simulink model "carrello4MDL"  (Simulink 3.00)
settings: Solver=ode45  SolverMode=SingleTasking  StartTime=0.0  StopTime=10.0  RelTol=1e-6  AbsTol=1e-7
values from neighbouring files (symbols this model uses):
  b1 = 2*1500*N/(m/sec)    (= 3000)    [carrello2.M]    (also in carrello3.M; carrello1.M; carrello4.M; carrello5.M)
  b2 = 2*1500*N/(m/sec)    (= 3000)    [carrello2.M]    (also in carrello3.M; carrello1.M; carrello4.M; carrello5.M)
  K = 0.8*1800*N/cm    (= 144000)    [carrello2.M]    (also in carrello3.M; carrello1.M; carrello4.M; carrello5.M)
  Kg = 1    [carrello2.M]    (also in carrello3.M; carrello1.M; carrello4.M = 10000000; carrello5.M)
  Kp = 2*1800*N/cm    (= 360000)    [carrello2.M]    (also in carrello3.M; carrello1.M; carrello4.M; carrello5.M)
  Ma = 3850*Kg    (= 3850)    [carrello2.M]    (also in carrello3.M; carrello1.M; carrello4.M; carrello5.M)
  mr = 2*134*Kg+524*Kg    (= 792)    [carrello2.M]    (also in carrello3.M; carrello1.M; carrello4.M; carrello5.M)
  R = 1    [carrello4.M]    (also in carrello5.M = 0.1; carrello6.M = 0.1)
  t1 = 0    [carrello4.M]
  t2 = 0    [carrello4.M]
  X_12_0 = -Mag/K    (= -0.26228125)    [carrello2.M]    (also in carrello3.M = 0; carrello1.M; carrello4.M = 0; carrello5.M = 0)
  X_20_0 = -(Mag+mrg)/Kp    (= -0.1264945)    [carrello2.M]    (also in carrello3.M = 0; carrello1.M; carrello4.M = 0; carrello5.M = 0)
  Xsdot = 0    [carrello3.M]    (also in carrello4.M; carrello5.M; carrello6.M)

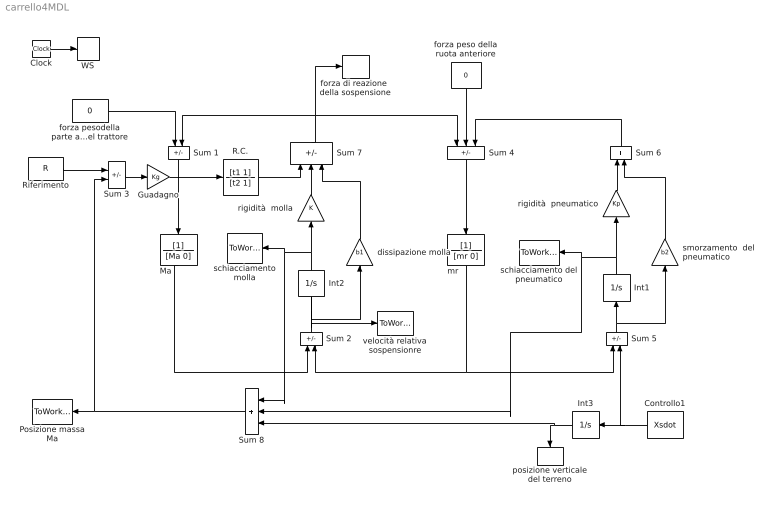
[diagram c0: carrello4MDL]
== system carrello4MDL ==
  Clock : Clock
  Controllo1 : Constant  Orientation=left  Value=Xsdot
  Guadagno : Gain  Gain=Kg  SaturateOnIntegerOverflow=on
  Int1 : Integrator  Orientation=up  ExternalReset=none  InitialConditionSource=internal  InitialCondition=X_20_0  LimitOutput=off  UpperSaturationLimit=inf  LowerSaturationLimit=-inf  ShowSaturationPort=off  ShowStatePort=off  AbsoluteTolerance=auto
  Int2 : Integrator  Orientation=up  ExternalReset=none  InitialConditionSource=internal  InitialCondition=X_12_0  LimitOutput=off  UpperSaturationLimit=inf  LowerSaturationLimit=-inf  ShowSaturationPort=off  ShowStatePort=off  AbsoluteTolerance=auto
  Int3 : Integrator  Orientation=left  ExternalReset=none  InitialConditionSource=internal  InitialCondition=X_20_0  LimitOutput=off  UpperSaturationLimit=inf  LowerSaturationLimit=-inf  ShowSaturationPort=off  ShowStatePort=off  AbsoluteTolerance=auto
  Ma : TransferFcn  Orientation=down  Numerator=[1]  Denominator=[Ma 0]
  Posizione massa Ma : ToWorkspace  VariableName=X_Ma  SampleTime=-1  SaveFormat=Matrix
  R.C. : TransferFcn  Numerator=[t1 1]  Denominator=[t2 1]
  Riferimento : Constant  Value=R
  Sum 1 : Sum  Orientation=down  Inputs=+-  SaturateOnIntegerOverflow=on
  Sum 2 : Sum  Orientation=up  Inputs=+-
  Sum 3 : Sum  Inputs=+-
  Sum 4 : Sum  Orientation=down  Inputs=++-
  Sum 5 : Sum  Orientation=up  Inputs=+-
  Sum 6 : Sum  Orientation=up  Inputs=++
  Sum 7 : Sum  Orientation=up  Inputs=-++
  Sum 8 : Sum  Orientation=left  Inputs=+++
  WS : ToWorkspace  VariableName=t  SampleTime=-1  SaveFormat=Matrix
  dissipazione molla : Gain  Orientation=up  Gain=b1  SaturateOnIntegerOverflow=on
  forza di reazione  della sospensione : ToWorkspace  VariableName=R  SampleTime=-1  SaveFormat=Matrix
  forza peso della ruota anteriore : Constant  Orientation=down  Value=0
  forza pesodella parte anteriore del trattore : Constant  Value=0
  mr : TransferFcn  Orientation=down  Numerator=[1]  Denominator=[mr 0]
  posizione verticale del terreno : ToWorkspace  VariableName=Xs  SampleTime=-1  SaveFormat=Matrix
  rigidità  molla : Gain  Orientation=up  Gain=K  SaturateOnIntegerOverflow=on
  rigidità  pneumatico : Gain  Orientation=up  Gain=Kp  SaturateOnIntegerOverflow=on
  schiacciamento del pneumatico : ToWorkspace  VariableName=X_20  SampleTime=-1  SaveFormat=Matrix
  schiacciamento molla : ToWorkspace  VariableName=X_12  SampleTime=-1  SaveFormat=Matrix
  smorzamento  del pneumatico : Gain  Orientation=up  Gain=b2  SaturateOnIntegerOverflow=on
  velocità relativa sospensionre : ToWorkspace  VariableName=vel_rel  SampleTime=-1  SaveFormat=Matrix
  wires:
  forza pesodella parte anteriore del trattore/1 -> Sum 1/1
  Sum 1/1 -> Ma/1
  forza peso della ruota anteriore/1 -> Sum 4/2
  Sum 4/1 -> mr/1
  mr/1 -> Sum 5/1, Sum 2/2
  Int1/1 -> rigidità  pneumatico/1, schiacciamento del pneumatico/1, Sum 8/2
  Sum 5/1 -> Int1/1, smorzamento  del pneumatico/1
  rigidità  pneumatico/1 -> Sum 6/1
  smorzamento  del pneumatico/1 -> Sum 6/2
  Sum 7/1 -> Sum 1/2, forza di reazione  della sospensione/1, Sum 4/1
  Sum 6/1 -> Sum 4/3
  Sum 2/1 -> velocità relativa sospensionre/1, Int2/1, dissipazione molla/1
  Int2/1 -> rigidità  molla/1, schiacciamento molla/1, Sum 8/1
  dissipazione molla/1 -> Sum 7/3
  rigidità  molla/1 -> Sum 7/2
  Ma/1 -> Sum 2/1
  Controllo1/1 -> Int3/1, Sum 5/2
  Int3/1 -> Sum 8/3, posizione verticale del terreno/1
  Clock/1 -> WS/1
  Riferimento/1 -> Sum 3/1
  Sum 8/1 -> Posizione massa Ma/1, Sum 3/2
  Sum 3/1 -> Guadagno/1
  Guadagno/1 -> R.C./1
  R.C./1 -> Sum 7/1
